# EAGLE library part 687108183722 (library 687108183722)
Wurth Elektronik WR-FPC Series 0.5mm Pitch 8 Way Horizontal SMT Female FPC Connector, Bottom Contact Source: Datasheet
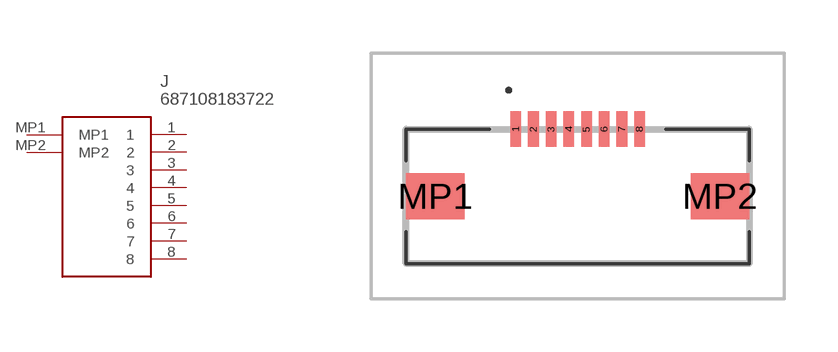
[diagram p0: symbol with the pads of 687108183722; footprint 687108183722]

Designator prefix J

## 687108183722 (Description: Wurth Elektronik WR-FPC Series 0.5mm Pitch 8 Way Horizontal SMT Female FPC Connector, Bottom Contact; Height: 1.3mm; Manufacturer_Name: Wurth Elektronik; Manufacturer_Part_Number: 687108183722; Mouser_Part_Number: 710-687108183722; Mouser_Price-Stock: https://www.mouser.co.uk/ProductDetail/Wurth-Elektronik/687108183722?qs=5aG0NVq1C4xXKc1RTH472A%3D%3D)  [687108183722]
1  1
2  2
3  3
4  4
5  5
6  6
7  7
8  8
MP1  MP1
MP2  MP2

## Footprint 687108183722 (pad centres in mm)
687108183722-2
smd 0.3 x 1: 1 -1.75,1.9; 2 -1.25,1.9; 3 -0.75,1.9; 4 -0.25,1.9; 5 0.25,1.9; 6 0.75,1.9; 7 1.25,1.9; 8 1.75,1.9
smd 1.65 x 1.3: MP1 -4.025,0; MP2 4.025,0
